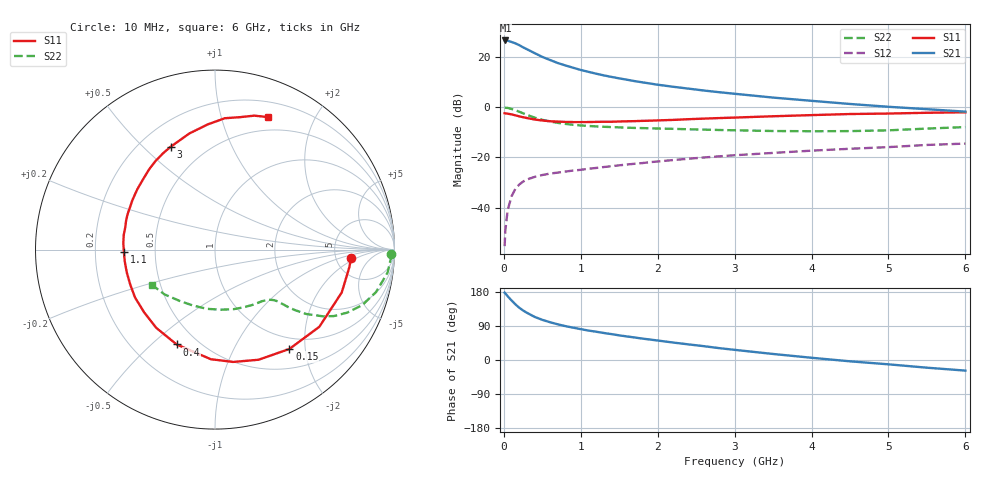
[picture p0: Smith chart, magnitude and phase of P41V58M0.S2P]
! SIEMENS Small Signal Semiconductors
! BFP182
! Si NPN RF Bipolar Junction Transistor in SOT143
! VCE = 1.5 V  IC = 8 mA
! Common Emitter S-Parameters:  March  1996
# GHz  S  MA  R  50
!  f  S11  S21  S12  S22
! GHz  MAG  ANG  MAG  ANG  MAG  ANG  MAG  ANG
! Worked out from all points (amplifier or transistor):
!   36 points, 10 MHz to 6 GHz, reference 50 ohm
!   highest |S21| = 26.7 dB at 20 MHz (marker M1)
!   |S21| within 3 dB of that: start of sweep to 267 MHz
!   unconditionally stable (mu >= 1): 1.2 GHz to 5.464 GHz
!   at 250 MHz: K = 0.30, MSG = 26.8 dB, |S12| = -29.6 dB
!   at 1.4 GHz: K = 1.07, MAG = 16.1 dB, |S12| = -23.5 dB
!   at 6 GHz: K = 0.96, MSG = 6.4 dB, |S12| = -14.5 dB
!   S11 on the Smith chart (normalised r, x): 10 MHz: 6.93, -1.60; 150 MHz: 0.80, -1.70; 400 MHz: 0.39, -0.60; 1.1 GHz: 0.33, -0.01; 3 GHz: 0.32, +0.61; 6 GHz: 0.35, +1.41
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0.01  0.7592 -3.7  21.31 177.8  0.0017 87.5  0.983 -1.5
0.02  0.7548 -7.5  21.52 175.7  0.0036 85.7  0.9803 -3.1
0.05  0.7455 -18.7  21.32 168.2  0.0089 82.5  0.9702 -7.6
0.1  0.7231 -36.5  20.07 157.2  0.0168 72.4  0.9276 -14.8
0.15  0.6915 -53.2  18.85 146.9  0.0236 64.9  0.8763 -20.7
0.2  0.66 -68.4  17.37 138.0  0.0288 59.0  0.8159 -25.5
0.25  0.6341 -80.8  15.7 130.7  0.033 54.9  0.7591 -29.2
0.3  0.6114 -92.1  14.39 124.6  0.0363 51.1  0.7077 -31.7
0.4  0.5701 -112.0  12.02 113.8  0.0409 46.1  0.6224 -35.2
0.5  0.5451 -126.9  10.12 106.0  0.0446 42.6  0.5622 -37.0
0.6  0.5272 -138.6  8.789 99.7  0.0477 41.0  0.5214 -38.1
0.7  0.5193 -149.2  7.646 94.2  0.0498 40.1  0.4896 -38.7
0.9  0.5077 -165.1  6.155 85.4  0.0548 40.1  0.4473 -39.8
1.1  0.5078 -178.4  5.095 77.7  0.0595 40.2  0.424 -41.4
1.5  0.5209 162.1  3.772 65.0  0.0696 40.7  0.3981 -45.4
1.8  0.536 149.4  3.148 56.5  0.0772 40.6  0.3848 -49.4
2.2  0.5604 135.7  2.568 46.1  0.0886 39.6  0.372 -56.0
3  0.6238 113.4  1.861 26.8  0.1106 35.5  0.3479 -72.5
3.5  0.6624 102.5  1.562 15.9  0.1231 32.4  0.3365 -84.6
4.5  0.7341 85.7  1.165 -3.5  0.1489 25.6  0.3351 -111.8
5.5  0.7775 73.7  0.917 -20.3  0.1775 18.5  0.3762 -138.5
6  0.7946 68.4  0.819 -28.0  0.1889 13.7  0.4034 -151.1
